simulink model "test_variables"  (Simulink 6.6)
settings: Solver=ode45  StartTime=0.0  StopTime=10.0  RelTol=1e-3
libraries: sltpda x3

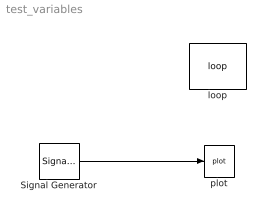
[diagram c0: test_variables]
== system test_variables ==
  Signal Generator : sltpda/Sources/Signal Generator  Tag=ao  SystemSampleTime=-1  nsecs=var1  fs=100  tsfcn=sin(2*pi*10*t)
  loop : sltpda/Parameters/loop  SystemSampleTime=-1  bname=<empty>  pname=<empty>  pvalues=0
  plot : sltpda/Sinks/plot  Tag=plot  Description=Plot an analysis object.  SystemSampleTime=-1  xscale=linear  yscale=linear
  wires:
  Signal Generator/1 -> plot/1
